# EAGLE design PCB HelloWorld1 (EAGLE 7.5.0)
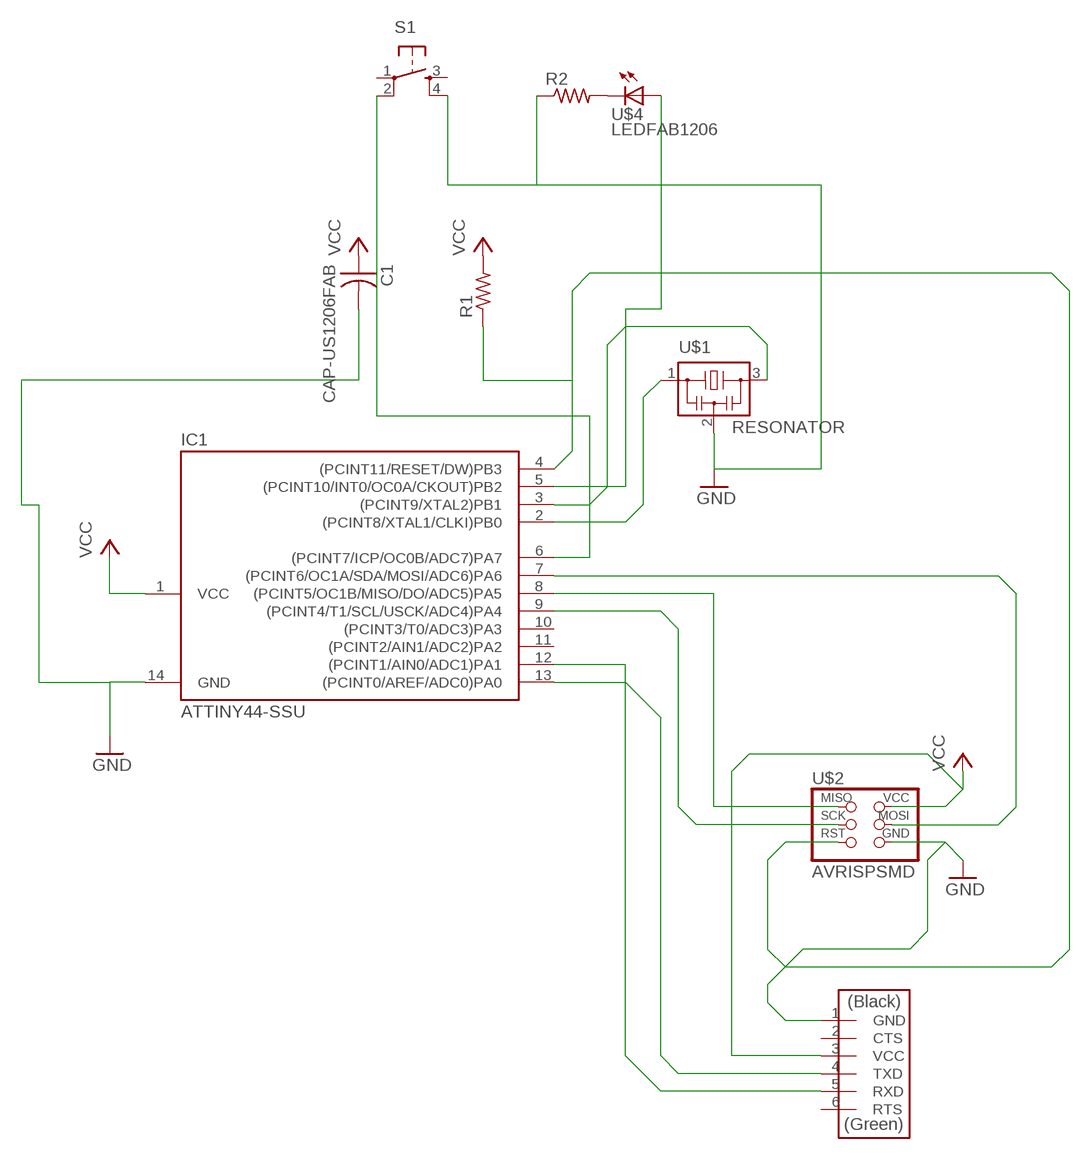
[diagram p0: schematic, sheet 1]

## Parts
C1  CAP-US1206FAB  [C1206FAB]
IC1  ATTINY44-SSU  [SOIC14]
R1  RES-US1206FAB  [R1206FAB]
R2  RES-US1206FAB  [R1206FAB]
S1  6MM_SWITCH6MM_SWITCH  [6MM_SWITCH]
U$1  RESONATOR  [EFOBM]
U$2  AVRISPSMD  [2X03SMD]
U$3  FTDI-SMD-HEADER  [1X06SMD]
U$4  LEDFAB1206  [LED1206FAB]

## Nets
GND: C1.2 IC1.14(GND) R2.1 S1.4(S1) U$1.2 U$2.6(GND) U$3.1(GND)
N$1: IC1.7((PCINT6/OC1A/SDA/MOSI/ADC6)PA6) U$2.4(MOSI)
N$2: IC1.3((PCINT9/XTAL2)PB1) U$1.3
N$3: IC1.2((PCINT8/XTAL1/CLKI)PB0) U$1.1
N$4: IC1.5((PCINT10/INT0/OC0A/CKOUT)PB2) U$4.1(A)
N$5: IC1.9((PCINT4/T1/SCL/USCK/ADC4)PA4) U$2.3(SCK)
N$6: IC1.4((PCINT11/RESET/DW)PB3) R1.1 U$2.5(RST)
N$7: IC1.8((PCINT5/OC1B/MISO/DO/ADC5)PA5) U$2.1(MISO)
N$8: IC1.13((PCINT0/AREF/ADC0)PA0) U$3.4(TXD)
N$9: IC1.12((PCINT1/AIN0/ADC1)PA1) U$3.5(RXD)
N$10: R2.2 U$4.2(C)
N$11: IC1.6((PCINT7/ICP/OC0B/ADC7)PA7) S1.2(P1)
VCC: C1.1 IC1.1(VCC) R1.2 U$2.2(VCC) U$3.3(VCC)
Unconnected: IC1.10((PCINT3/T0/ADC3)PA3) IC1.11((PCINT2/AIN1/ADC2)PA2) S1.1(P) S1.3(S) U$3.2(CTS) U$3.6(RTS)

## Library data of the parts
C1 = fab:CAP-US
IC1 = fab:ATTINY44
R1 R2 = fab:RES-US: Resistor (US Symbol)
S1 = fab:6MM_SWITCH: OMRON SWITCH
U$1 = fab:RESONATOR
U$2 = fab:AVRISP
U$3 = fab:FTDI-SMD-HEADER
U$4 = fab:LED: LED

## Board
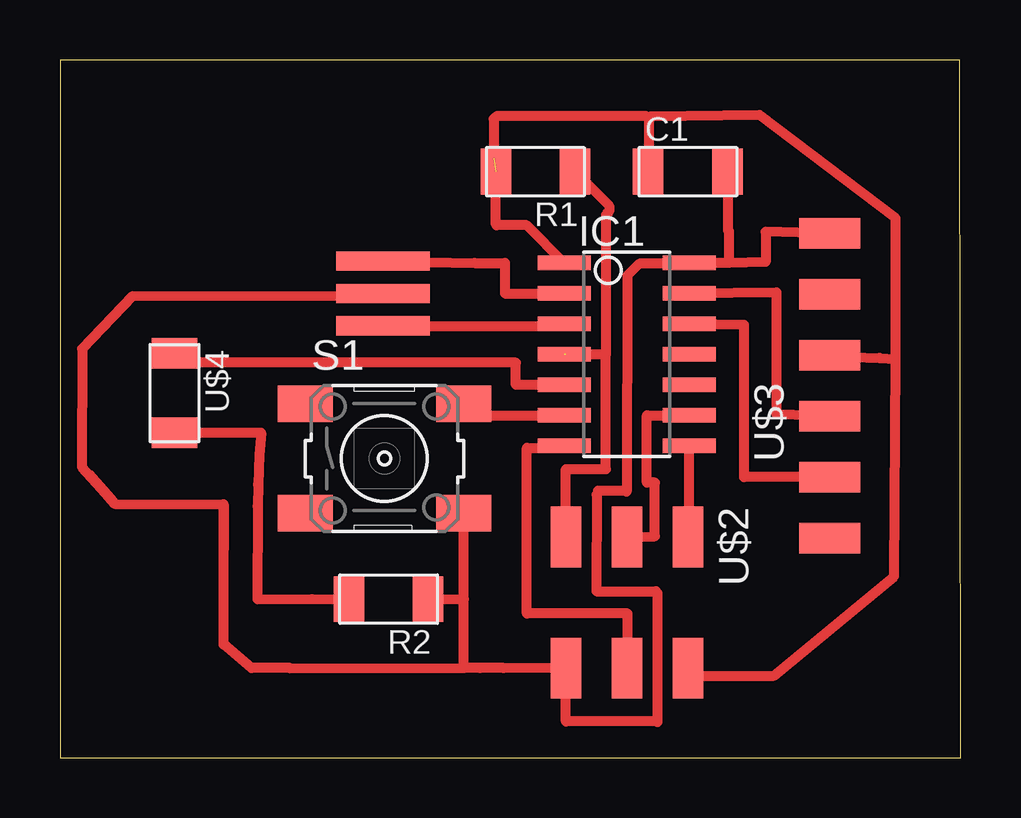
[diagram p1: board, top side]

Size 37.53 x 29.1 mm. Coordinates in mm from the lower left corner, seen from the top.
Outline: 0,0.01 37.53,0 37.49,29.08 0.02,29.1 0,0.01
Copper layers 1: Top 0.035mm
Design rules "default *": minimum track width 10mil, minimum drill 0.8mm, track to track 0.42mm, track to pad 0.42mm, pad to pad 0.42mm, via to via 0.42mm, smd to smd 8mil, copper to edge 1mil, drill to drill 1mil, minimum pad ring 10mil, minimum via ring 8mil, stop-mask expansion 4mil, vias tented up to drill 0mil, thermal gap 10mil

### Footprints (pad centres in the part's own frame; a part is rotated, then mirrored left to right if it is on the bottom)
C1206FAB = smd 1.27 x 1.905: 1 -1.651,0; 2 1.651,0
SOIC14 = smd 0.61 x 2.21: 1 -3.81,-2.603; 2 -2.54,-2.603; 3 -1.27,-2.603; 4 0,-2.603; 5 1.27,-2.603; 6 2.54,-2.603; 7 3.81,-2.603; 8 3.81,2.603; 9 2.54,2.603; 10 1.27,2.603; 11 0,2.603; 12 -1.27,2.603; 13 -2.54,2.603; 14 -3.81,2.603
R1206FAB = smd 1.27 x 1.905: 1 -1.651,0; 2 1.651,0
6MM_SWITCH = smd 2.286 x 1.524: 1 -3.302,2.286; 2 3.302,2.286; 3 -3.302,-2.286; 4 3.302,-2.286
EFOBM = smd 0.8 x 3.9: 1 -1.35,0; 2 0,0; 3 1.35,0
2X03SMD = smd 2.54 x 1.27: 1 -2.54,2.54; 2 2.92,2.54; 3 -2.54,0; 4 2.92,0; 5 -2.54,-2.54; 6 2.92,-2.54
1X06SMD = smd 2.54 x 1.27: 1 0,6.35; 2 0,3.81; 3 0,1.27; 4 0,-1.27; 5 0,-3.81; 6 0,-6.35
LED1206FAB = smd 1.27 x 1.905: 1 -1.651,0; 2 1.651,0

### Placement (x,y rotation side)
C1  26.16,24.45 0 top
IC1  23.62,16.83 270 top
R1  19.81,24.45 180 top
R2  13.69,6.62 180 top
S1  13.52,12.49 0 top
U$1  13.46,19.37 270 top
U$2  23.62,6.67 270 top
U$3  32.07,15.52 0 top
U$4  4.77,15.21 270 top

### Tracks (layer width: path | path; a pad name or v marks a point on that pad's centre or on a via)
GND
  Top 0.406: U$3.1 29.4,21.94 29.4,20.67 27.87,20.64 | 27.87,20.64 IC1.14 26.19,20.61 24.14,20.61 23.64,20.11 23.61,11.11 23.61,11.13 22.42,11.13 22.36,10.98 22.35,7.02 22.35,6.95 24.83,6.95 24.89,6.87 24.89,1.49 24.86,1.53 21.09,1.53 21.08,1.53 U$2.6 18.49,3.75 17.51,3.75 16.83,3.75 | 16.83,3.75 16.83,6.62 | 16.83,6.62 S1.4 | R2.1 16.83,6.62 | C1.2 27.83,24.43 27.83,22 27.87,21.95 27.87,20.64 | U$1.2 13.33,19.23 3.03,19.25 0.92,17.06 0.92,12.14 2.14,10.78 1.19,11.83 2.28,10.6 6.82,10.58 | 16.83,3.75 9.57,3.74 9.59,3.75 7.98,3.75 6.82,4.73 6.82,10.58 | 6.82,10.58 6.82,8.67
N$1
  Top 0.406: U$2.4 23.65,3.75 23.65,6.03 19.45,6.03 19.45,12.93 21.02,12.93 IC1.7
N$2
  Top 0.406: U$1.3 21.02,18.02 IC1.3
N$3
  Top 0.406: U$1.1 17.27,20.64 18.54,20.64 18.54,19.37 IC1.2
N$4
  Top 0.406: IC1.5 19,15.56 19,16.48 4.73,16.48 U$4.1
N$5
  Top 0.406: U$2.3 24.79,9.25 24.79,11.48 | IC1.9 24.49,14.29 24.45,14.29 24.45,11.48 24.79,11.48 | 24.79,11.48 24.8,11.48
N$6  (1 unrouted)
  Top 0.406: U$2.5 21.08,12.05 22.75,12.05 22.75,16.83 | 22.75,16.83 21.08,16.83 | R1.1 22.88,23.03 22.88,22.78 22.75,22.65 22.75,16.83
N$7
  Top 0.406: U$2.1 26.22,9.21 IC1.8
N$8
  Top 0.406: U$3.4 29.86,14.32 29.86,19.4 IC1.13
N$9
  Top 0.406: U$3.5 28.5,11.71 28.5,18.06 IC1.12
N$10
  Top 0.406: U$4.2 8.38,13.56 8.31,12.63 8.26,11.4 8.26,11.41 8.23,10.49 8.22,6.62 10.5,6.63 R2.2
N$11
  Top 0.406: S1.2 16.85,14.27 18.95,14.28 IC1.6
VCC  (1 unrouted)
  Top 0.406: IC1.1 19.44,22.21 18.19,22.21 18.16,22.24 R1.2 | C1.1 24.56,24.5 24.56,26.64 | 24.56,26.64 24.56,26.73 29.15,26.81 34.82,22.5 34.82,16.64 | 24.56,26.64 24.44,26.75 18.19,26.75 18.07,26.64 18.07,25 | U$3.3 31.89,16.75 34.14,16.68 34.82,16.64 | U$2.2 26.47,3.43 29.75,3.43 34.76,7.57 34.82,16.64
